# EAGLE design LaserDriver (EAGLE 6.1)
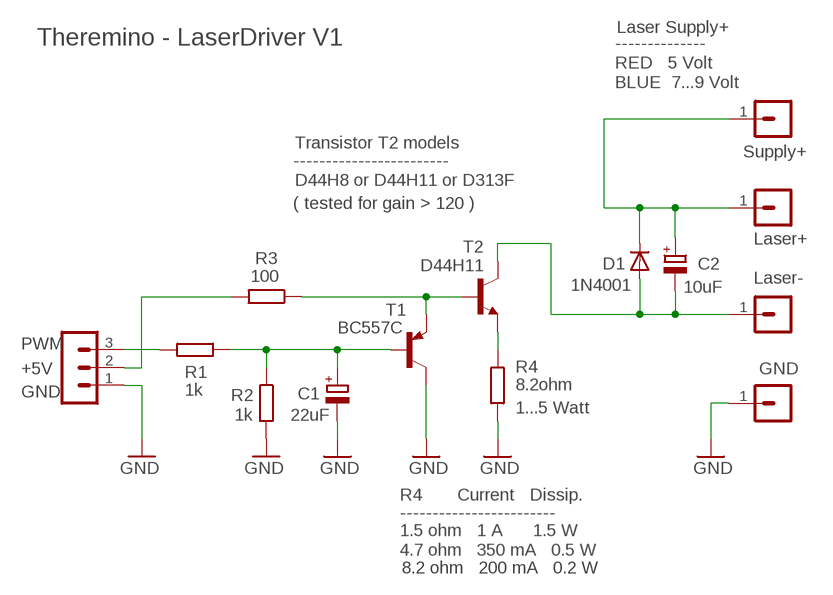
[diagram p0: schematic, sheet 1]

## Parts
C1  22uF  CPOL-EUE2-5B  [E2-5B]
C2  10uF  CPOL-EUE2-5B  [E2-5B]
D1  1N4001  DIODE-DO34-7  [DO34-7]
R1  1k  R-EU_0204/5  [0204/5]
R2  1k  R-EU_0204/5  [0204/5]
R3  100  R-EU_0204/5  [0204/5]
R4  8.2ohm  R-EU_0309/12  [0309/12]
SV1  GND  MA01-1  [MA01-1]
SV2  Laser-  MA01-1  [MA01-1]
SV3  Laser+  MA01-1  [MA01-1]
SV4  Supply+  MA01-1  [MA01-1]
SV5  PWM  MA03-1N  [MA03-1]
T1  BC557C  -PNP-TO92-CBE  [TO92-CBE]
T2  D44H11  -NPN-TO220  [TO220]

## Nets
GND: C1.- R2.2 R4.2 SV1.1 SV5.1 T1.C
N$1: C1.+ R1.1 R2.1 T1.B
N$2: R1.2 SV5.3
N$3: R3.2 SV5.2
N$4: C2.- D1.A SV2.1 T2.2(C)
N$5: C2.+ D1.C SV3.1 SV4.1
N$6: R4.1 T2.3(E)
N$7: R3.1 T1.E T2.1(B)

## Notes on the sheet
- Laser Supply+
- Theremino - LaserDriver V1 | --------------
- RED   5 Volt
- BLUE  7...9 Volt
- Transistor T2 models
- ------------------------
- D44H8 or D44H11 or D313F
- ( tested for gain > 120 )
- R4       Current   Dissip.
- ------------------------
- 1.5 ohm   1 A      1.5 W
- 4.7 ohm   350 mA   0.5 W
- 8.2 ohm   200 mA   0.2 W

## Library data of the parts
C1 C2 = 00-LIVIO:CPOL-EU: POLARIZED CAPACITOR, European symbol
D1 = 00-LIVIO:DIODE-: DIODE
R1-R3 = 00-LIVIO:R-EU_: RESISTOR, European symbol
R4 = 00-LIVIO:R-EU_: RESISTOR, European symbol; POWER: 1...5 Watt
SV1-SV4 = 03-con-lstb-M:MA01-1: PIN HEADER
SV5 = 03-con-lstb-M:MA03-1: PIN HEADER; 5V: +5V; GND: GND
T1 = 00-LIVIO:*-PNP-: PNP Transistror
T2 = 00-LIVIO:*-NPN-: NPN Transistror

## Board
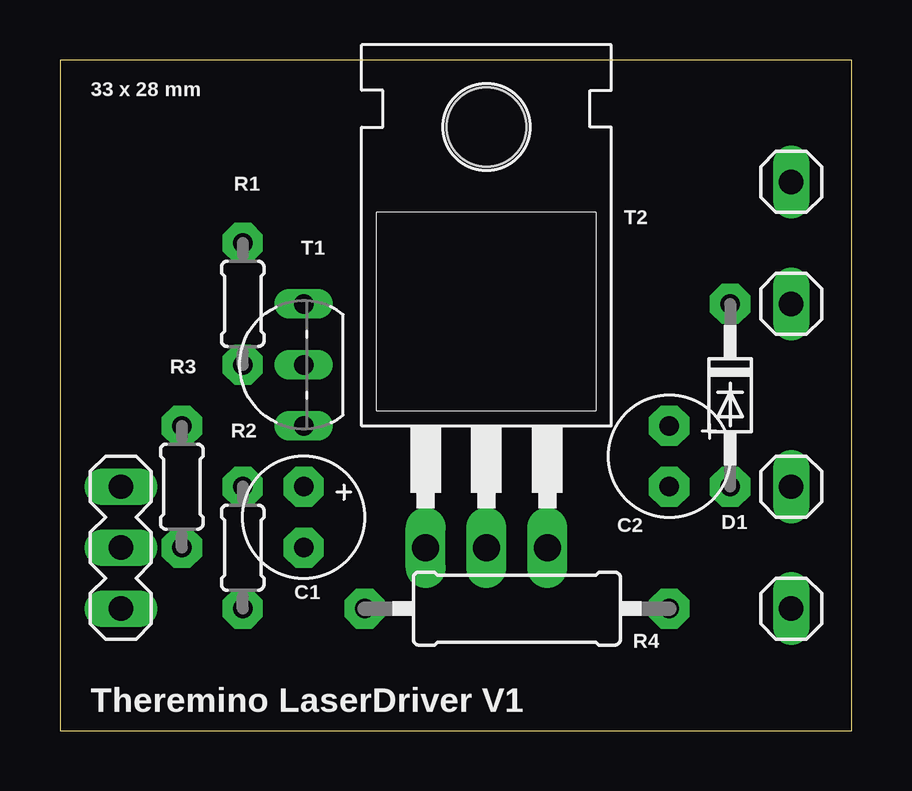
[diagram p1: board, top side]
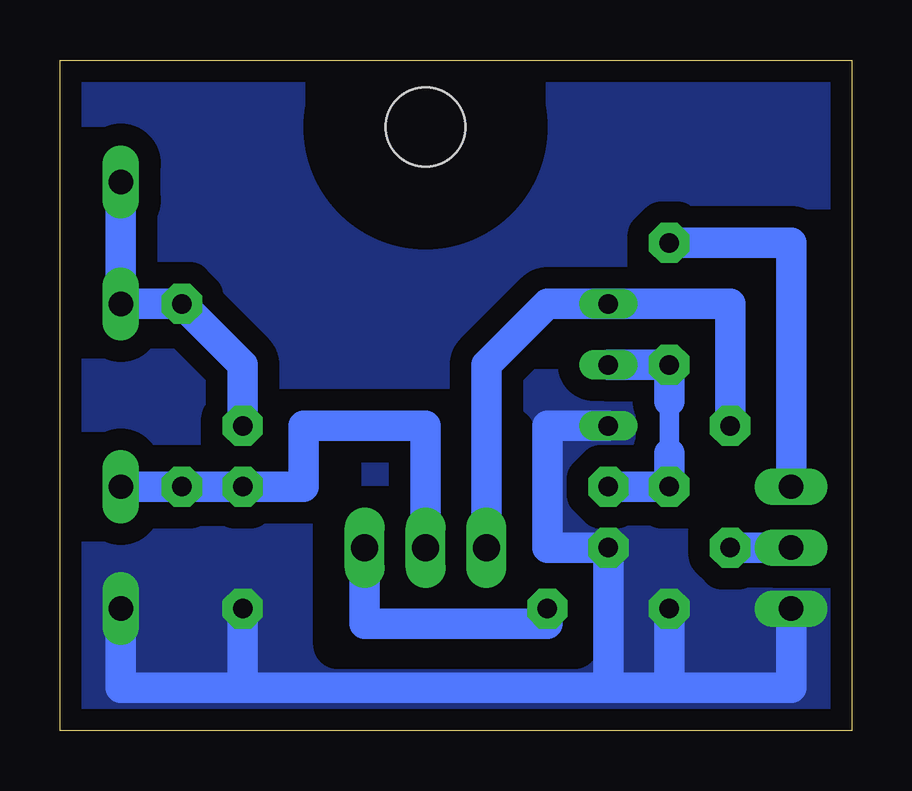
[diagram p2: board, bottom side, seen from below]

Size 33.02 x 27.94 mm. Coordinates in mm from the lower left corner, seen from the top.
Outline: 0,0 33.02,0 33.02,27.94 0,27.94 0,0
Copper layers (1*16): Top 0.035mm / dielectric 1.5mm / Bottom 0.035mm
Design rules: minimum track width 10mil, minimum drill 0.6mm, track to track 8mil, track to pad 8mil, pad to pad 8mil, via to via 8mil, smd to smd 8mil, copper to edge 31mil, drill to drill 8mil, minimum pad ring 5mil, minimum via ring 8mil, stop-mask expansion 4mil, vias tented up to drill 0mil, thermal gap 47mil
bRestrict: 5 lines

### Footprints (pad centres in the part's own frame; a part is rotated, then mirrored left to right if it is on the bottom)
E2-5B = drill 0.813 pad 1.676 octagon: + -1.27,0; - 1.27,0
DO34-7 = drill 0.813 pad 1.676 octagon: A 3.81,0; C -3.81,0
0204/5 = drill 0.813 pad 1.676 octagon: 1 -2.54,0; 2 2.54,0
0309/12 = drill 0.813 pad 1.676 octagon: 1 -6.35,0; 2 6.35,0
MA01-1 = drill 1.016 long: 1 0,0
MA03-1 = drill 1.016 long: 1 -2.54,0; 2 0,0; 3 2.54,0
TO92-CBE = drill 0.813 long: B 0,0; C -2.54,0; E 2.54,0
TO220 = drill 1.118 long: 1 -2.54,-6.35; 2 0,-6.35; 3 2.54,-6.35 | hole 3.302: 0,11.176

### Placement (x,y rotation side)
C1  10.16,8.89 270 top
C2  25.4,11.43 270 top
D1  27.94,13.97 270 top
R1  7.62,17.78 90 top
R2  7.62,7.62 270 top
R3  5.08,10.16 270 top
R4  19.05,5.08 0 top
SV1  30.48,5.08 0 top
SV2  30.48,10.16 0 top
SV3  30.48,17.78 0 top
SV4  30.48,22.86 0 top
SV5  2.54,7.62 90 top
T1  10.16,15.24 90 top
T2  17.78,13.97 0 top

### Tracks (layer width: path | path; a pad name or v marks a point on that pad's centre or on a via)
GND
  Bottom 1.27: 25.4,1.78 30.48,1.78 SV1.1 | 25.4,1.78 10.16,1.78 | T1.C 12.7,12.7 12.7,7.62 C1.- 10.16,1.78 | 7.62,1.78 2.54,1.78 SV5.1 | R2.2 7.62,1.78 | 10.16,1.78 7.62,1.78 | R4.2 25.4,1.78
  pour Bottom (isolate 0.9, rank 6, no thermals): -1,-1 34.02,-1 34.02,28.94 -1,28.94
N$1
  Bottom 0.813: 7.62,11.56 7.62,13.72
  Bottom 1.27: C1.+ R2.1 7.62,11.56 | 7.62,13.72 R1.1 T1.B
N$2
  Bottom 1.27: R1.2 2.54,20.32 SV5.3
N$3
  Bottom 1.27: SV5.2 R3.2
N$4
  Bottom 1.27: T2.2 17.78,12.7 22.86,12.7 22.86,10.16 C2.- D1.A SV2.1
N$5
  Bottom 1.27: C2.+ 25.4,15.24 D1.C SV3.1 SV4.1
N$6
  Bottom 1.27: T2.3 20.32,4.45 12.7,4.45 R4.1
N$7
  Bottom 1.27: T2.1 15.24,15.24 12.7,17.78 T1.E 5.08,17.78 R3.1

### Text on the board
tNames: 33 x 28 mm | Theremino LaserDriver V1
